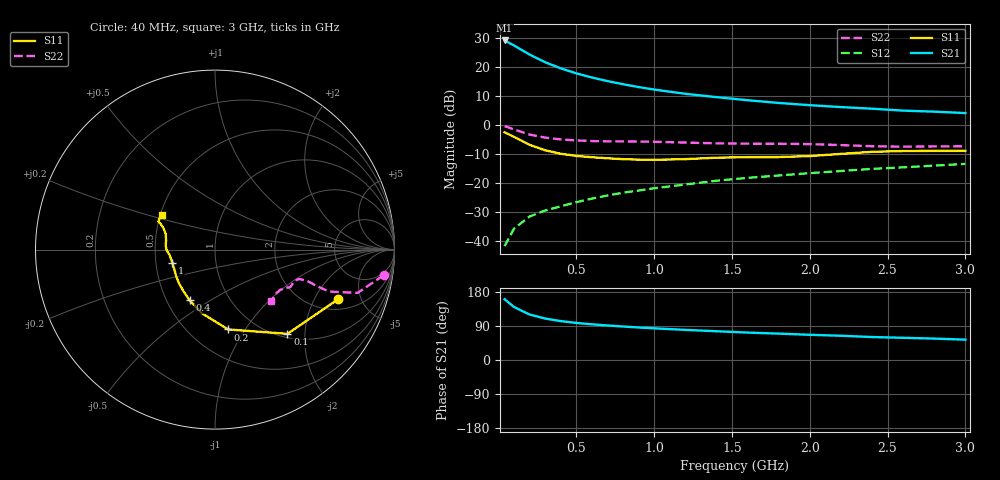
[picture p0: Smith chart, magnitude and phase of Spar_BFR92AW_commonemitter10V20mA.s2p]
! Filename:  BFR92AWJ.S2P  Version:  4.0
! NXP part #: BFR92AW  Date: Jun 1994
! Bias condition: Vce=10V, Ic=20mA
#  MHz  S  MA  R  50
! Freq  S11  S21  S12  S22  !GUM [dB]
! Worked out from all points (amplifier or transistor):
!   21 points, 40 MHz to 3 GHz, reference 50 ohm
!   highest |S21| = 29.1 dB at 40 MHz (marker M1)
!   |S21| within 3 dB of that: start of sweep to 140.7 MHz
!   unconditionally stable (mu >= 1): 519.7 MHz to end of sweep
!   at 300 MHz: K = 0.81, MSG = 25.6 dB, |S12| = -29.6 dB
!   at 1 GHz: K = 1.12, MAG = 15.0 dB, |S12| = -21.9 dB
!   at 3 GHz: K = 1.10, MAG = 6.9 dB, |S12| = -13.5 dB
!   S11 on the Smith chart (normalised r, x): 40 MHz: 2.59, -3.17; 100 MHz: 1.07, -1.63; 200 MHz: 0.75, -0.84; 400 MHz: 0.65, -0.41; 1 GHz: 0.61, -0.09; 3 GHz: 0.51, +0.23
40  0.74 -21.9  28.61 160.4  0.008 78.7  0.95 -8.7
100  0.619 -49.3  23.46 140.0  0.016 69.0  0.83 -16.9
200  0.451 -80.6  16.35 120.0  0.026 63.4  0.677 -20.2
300  0.363 -101.3  12.06 109.4  0.033 63.6  0.6 -19.7
400  0.316 -116.6  9.447 102.6  0.039 65.5  0.559 -19.0
500  0.29 -127.5  7.735 97.9  0.046 67.0  0.536 -18.8
600  0.275 -136.8  6.559 94.2  0.053 69.0  0.524 -18.9
700  0.264 -144.1  5.686 91.1  0.06 70.3  0.518 -19.0
800  0.255 -151.0  5.019 88.4  0.067 71.4  0.516 -19.0
900  0.25 -157.3  4.489 85.8  0.073 72.0  0.513 -19.0
1000  0.248 -163.1  4.06 83.6  0.08 72.5  0.508 -19.0
1200  0.255 -173.3  3.431 79.5  0.093 73.4  0.493 -19.5
1400  0.27 -179.8  3.002 75.9  0.108 74.1  0.478 -21.3
1600  0.276 175.2  2.657 72.4  0.121 74.2  0.471 -24.2
1800  0.277 169.6  2.383 69.6  0.133 74.9  0.47 -26.0
2000  0.288 162.4  2.18 66.5  0.146 75.2  0.464 -27.0
2200  0.314 156.9  2.022 64.0  0.159 75.4  0.446 -28.4
2400  0.341 154.2  1.896 60.6  0.173 75.6  0.426 -32.0
2600  0.352 153.7  1.756 58.6  0.184 75.4  0.418 -36.8
2800  0.354 151.3  1.686 56.5  0.197 76.1  0.423 -40.3
3000  0.354 146.8  1.593 53.7  0.211 76.3  0.426 -42.4
